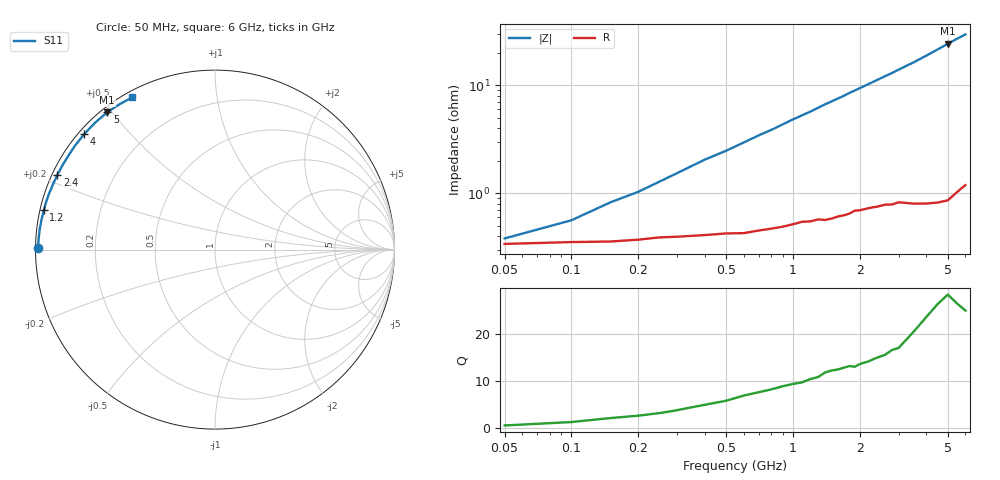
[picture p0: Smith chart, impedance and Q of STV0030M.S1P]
! SIEMENS Discrete & RF Semiconductors
! BA892
! Si PIN Diode in SCD-80
! IF = 30 mA
! S-Parameters:  September  1997
# GHz  S  MA  R  50
!  f  S11
! GHz  MAG  ANG
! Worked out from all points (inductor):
!   34 points, 50 MHz to 6 GHz, reference 50 ohm
!   read as one part to ground: L = 787 pH near 250 MHz
!   highest Q = 26.4 at 5 GHz (marker M1), where L = 774 pH
!   S11 on the Smith chart (normalised r, x): 50 MHz: 0.01, +0.00; 1.2 GHz: 0.01, +0.11; 2.4 GHz: 0.02, +0.22; 4 GHz: 0.02, +0.38; 5 GHz: 0.02, +0.49; 6 GHz: 0.02, +0.59
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0.05  0.9865 179.6
0.1  0.986 179.0
0.15  0.9858 178.3
0.2  0.9853 177.8
0.4  0.9838 175.4
0.5  0.9832 174.4
0.6  0.9831 173.3
0.7  0.9822 172.2
0.8  0.9815 171.2
1  0.9798 169.0
1.2  0.9786 167.0
1.3  0.9777 165.9
1.4  0.978 164.8
1.6  0.9765 162.8
1.7  0.9759 161.8
1.8  0.9751 160.7
1.9  0.9736 159.7
2.2  0.9724 156.7
2.4  0.9718 154.7
2.6  0.9708 152.7
2.8  0.9709 150.8
3  0.9699 148.7
3.5  0.9715 143.8
4  0.9723 138.6
4.5  0.9727 133.3
5  0.9726 128.1
5.5  0.9688 123.1
6  0.9654 118.6
